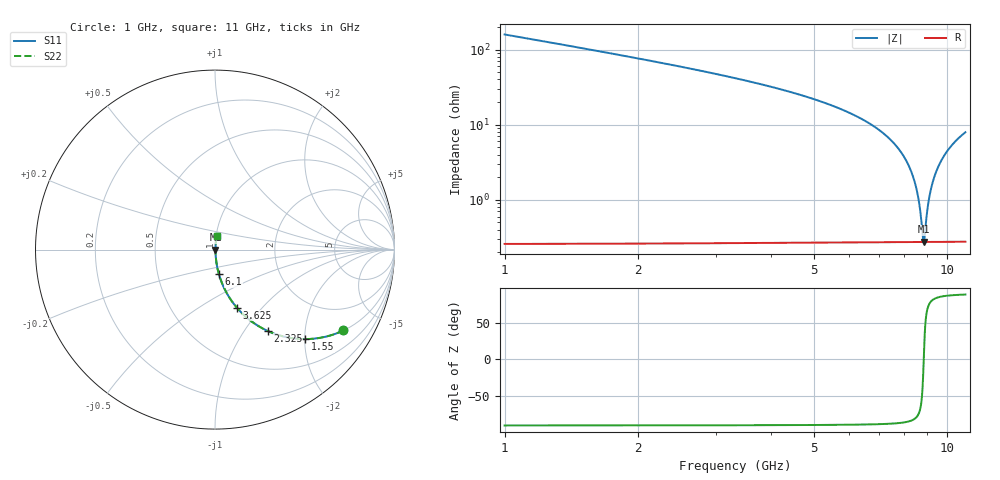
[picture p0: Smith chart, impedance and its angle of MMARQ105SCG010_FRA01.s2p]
! MMARQ105SCG010_FRA01  S-PARAMETER MODEL  ( General Type )
! Model Generated by TAIYO YUDEN Corporation (http://www.ty-top.com)
! Version 1.0
! TAIYO YUDEN Control No. 200326
! Copyright(c) 2020 TAIYO YUDEN CO.,LTD. All Rights Reserved.
! Product Description (link to TY-COMPAS)
! https://ds.yuden.co.jp/TYCOMPAS/or/detail?pn=MMARQ105SCG010BFRA01&u=M
! Products Name : Multilayer Ceramic Capacitors
! Characteristics :
!  Capacitance : 1 pF , Rated Voltage : 250V , TCC : CG / C0G
!  Case Size : 1.0 x 0.5 / 0.039 x 0.02 [mm/inch] , Thickness : 0.5 / 0.02 [mm/inch]
!  (Conditions: Temperature = 25 degC , DC Bias Current/Voltage = 0A / 0V)
! External Node Assignments :
!  1  o---| |---o  2
! GND o---------o GND
! Frequency Range : 1GHz  -  11GHz  [ 401 STEP ]
# MHz S RI R 50
! Freq[MHz].  S11 Real  S11 Imag  S21 Real  S21 Imag  S12 Real  S12 Imag  S22 Real  S22 Imag
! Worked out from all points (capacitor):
!   401 points, 1 GHz to 11 GHz, reference 50 ohm
!   read as one part in series: C = 990 fF near 1.05 GHz
!   lowest |Z| = 277 mohm at 8.85 GHz (marker M1)
!   series resonance near 8.856 GHz, so ESL is about 330 pH
!   S11 on the Smith chart (normalised r, x): 1 GHz: 1.01, -3.18; 1.55 GHz: 1.01, -2.01; 2.325 GHz: 1.01, -1.29; 3.625 GHz: 1.01, -0.74; 6.1 GHz: 1.01, -0.28; 11 GHz: 1.01, +0.16
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1000  0.7156 -0.4503  0.2844 0.4503  0.2844 0.4503  0.7156 -0.4503
1550  0.5028 -0.4987  0.4972 0.4987  0.4972 0.4987  0.5028 -0.4987
2325  0.2939 -0.4535  0.7061 0.4535  0.7061 0.4535  0.2939 -0.4535
2675  0.2309 -0.419  0.7691 0.419  0.7691 0.419  0.2309 -0.419
3625  0.1218 -0.3234  0.8782 0.3234  0.8782 0.3234  0.1218 -0.3234
4350  0.075 -0.2587  0.925 0.2587  0.925 0.2587  0.075 -0.2587
6000  0.0231 -0.1412  0.9769 0.1412  0.9769 0.1412  0.0231 -0.1412
6100  0.0214 -0.1352  0.9786 0.1352  0.9786 0.1352  0.0214 -0.1352
7000  0.01 -0.0851  0.99 0.0851  0.99 0.0851  0.01 -0.0851
7675  0.00543 -0.0517  0.9946 0.0517  0.9946 0.0517  0.00543 -0.0517
8100  0.00378 -0.0322  0.9962 0.0322  0.9962 0.0322  0.00378 -0.0322
8425  0.00307 -0.018  0.9969 0.018  0.9969 0.018  0.00307 -0.018
8625  0.00284 -0.00954  0.9972 0.00954  0.9972 0.00954  0.00284 -0.00954
8800  0.00275 -0.00229  0.9972 0.00229  0.9972 0.00229  0.00275 -0.00229
8850  0.00275 -0.000242  0.9973 0.000242  0.9973 0.000242  0.00275 -0.000242
8900  0.00275 0.00179  0.9972 -0.00179  0.9972 -0.00179  0.00275 0.00179
9025  0.0028 0.00683  0.9972 -0.00683  0.9972 -0.00683  0.0028 0.00683
9100  0.00285 0.00982  0.9972 -0.00982  0.9972 -0.00982  0.00285 0.00982
9350  0.00314 0.0196  0.9969 -0.0196  0.9969 -0.0196  0.00314 0.0196
9625  0.00366 0.0301  0.9963 -0.0301  0.9963 -0.0301  0.00366 0.0301
9975  0.00461 0.043  0.9954 -0.043  0.9954 -0.043  0.00461 0.043
11000  0.00897 0.0784  0.991 -0.0784  0.991 -0.0784  0.00897 0.0784
